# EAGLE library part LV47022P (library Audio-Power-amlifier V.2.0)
SANYO 4 x48W - Chanel BTL Power Amplifier
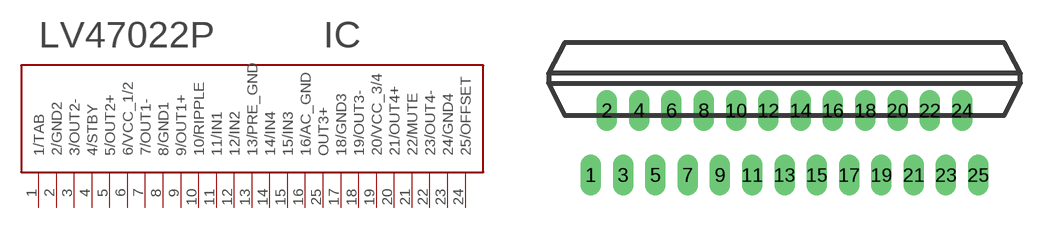
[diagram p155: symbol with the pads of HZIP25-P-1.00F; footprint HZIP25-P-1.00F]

Designator prefix IC

## LV47022P  [HZIP25-P-1.00F]
1  1/TAB
2  2/GND2  pwr
3  3/OUT2-  out
4  4/STBY  in
5  5/OUT2+  out
6  6/VCC_1/2  pwr
7  7/OUT1-  out
8  8/GND1  pwr
9  9/OUT1+  out
10  10/RIPPLE
11  11/IN1  in
12  12/IN2  in
13  13/PRE_GND  pwr
14  14/IN4  in
15  15/IN3  in
16  16/AC_GND  pwr
17  18/GND3  pwr
18  19/OUT3-  out
19  20/VCC_3/4  pwr
20  21/OUT4+  out
21  22/MUTE  in
22  23/OUT4-  out
23  24/GND4  pwr
24  25/OFFSET  in
25  OUT3+  out

## Footprint HZIP25-P-1.00F (pad centres in mm)
HZIP25-P-1.00F
drill 0.5 pad 1.27 long: 1 -12,-4; 2 -11,0; 3 -10,-4; 4 -9,0; 5 -8,-4; 6 -7,0; 7 -6,-4; 8 -5,0; 9 -4,-4; 10 -3,0; 11 -2,-4; 12 -1,0; 13 0,-4; 14 1,0; 15 2,-4; 16 3,0; 17 4,-4; 18 5,0; 19 6,-4; 20 7,0; 21 8,-4; 22 9,0; 23 10,-4; 24 11,0; 25 12,-4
